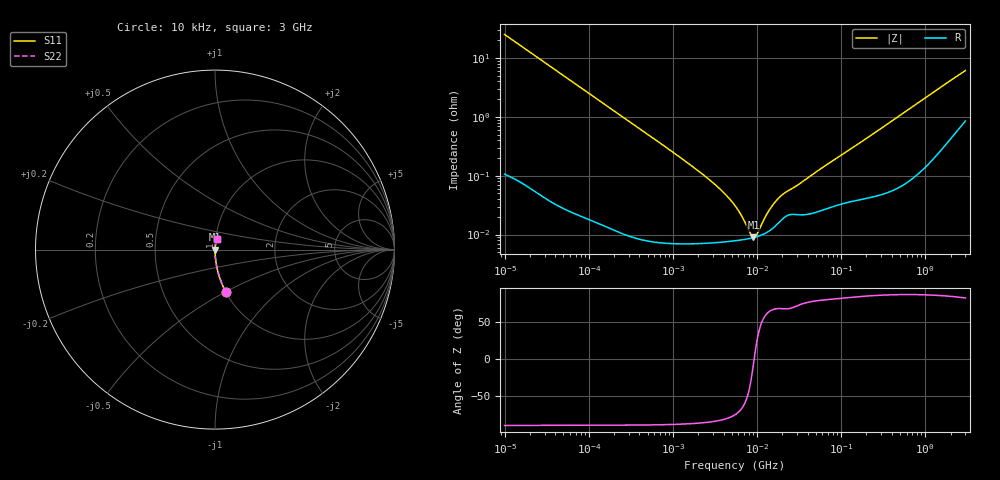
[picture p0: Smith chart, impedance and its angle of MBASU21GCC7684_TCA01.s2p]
! MBASU21GCC7684_TCA01  S-PARAMETER MODEL  ( Standard Model )
! Model Generated by TAIYO YUDEN Corporation (http://www.ty-top.com)
! Version 1.0
! TAIYO YUDEN Control No. 220601
! Copyright(c) 2014 TAIYO YUDEN CO.,LTD. All Rights Reserved.
! Product Description (link to TY-COMPAS)
! https://ds.yuden.co.jp/TYCOMPAS/or/detail?pn=MBASU21GCC7684KTCA01&u=M
! Products Name : Multilayer Ceramic Capacitors
! Characteristics :
!  Capacitance : 0.68 [uF] , Rated Voltage : 50 [V] , TCC : X7S
!  Case Size : 2.0 x 1.25 / 0.079 x 0.049 [mm/inch] , Thickness : 1.25 / 0.049 [mm/inch]
!  (Conditions: Temperature = 25 [degC] , DC Bias Voltage = 0 [V])
! External Node Assignments :
!  1  o---| |---o  2
! GND o---------o GND
! Frequency Range : 10kHz  -  3GHz  [ 401 STEP ]
# MHZ S RI R 50
! Freq[MHz].  S11 Real  S11 Imag  S21 Real  S21 Imag  S12 Real  S12 Imag  S22 Real  S22 Imag
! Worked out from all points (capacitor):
!   401 points, 10 kHz to 3 GHz, reference 50 ohm
!   read as one part in series: C = 631 nF near 10.65 kHz
!   lowest |Z| = 8.95 mohm at 9.071 MHz (marker M1)
!   series resonance near 9.261 MHz, so ESL is about 470 pH
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0.01  0.0605 -0.2364  0.9395 0.2364  0.9395 0.2364  0.0605 -0.2364
0.02575  0.01 -0.0971  0.99 0.0971  0.99 0.0971  0.01 -0.0971
0.082683  0.00114 -0.0306  0.9989 0.0306  0.9989 0.0306  0.00114 -0.0306
0.683653  8.65e-05 -0.00371  0.9999 0.00371  0.9999 0.00371  8.65e-05 -0.00371
1.601553  7.18e-05 -0.00154  0.9999 0.00154  0.9999 0.00154  7.18e-05 -0.00154
2.737278  7.24e-05 -0.000846  0.9999 0.000846  0.9999 0.000846  7.24e-05 -0.000846
4.124064  7.54e-05 -0.000492  0.9999 0.000492  0.9999 0.000492  7.54e-05 -0.000492
5.477226  7.86e-05 -0.0003  0.9999 0.0003  0.9999 0.0003  7.86e-05 -0.0003
6.617858  8.14e-05 -0.000187  0.9999 0.000187  0.9999 0.000187  8.14e-05 -0.000187
8.252149  8.6e-05 -6.33e-05  0.9999 6.33e-05  0.9999 6.33e-05  8.6e-05 -6.33e-05
9.070798  8.87e-05 -1.13e-05  0.9999 1.13e-05  0.9999 1.13e-05  8.87e-05 -1.13e-05
9.6612  9.09e-05 2.32e-05  0.9999 -2.32e-05  0.9999 -2.32e-05  9.09e-05 2.32e-05
10.29003  9.34e-05 5.8e-05  0.9999 -5.8e-05  0.9999 -5.8e-05  9.34e-05 5.8e-05
13.66633  0.000113 0.000219  0.9999 -0.000219  0.9999 -0.000219  0.000113 0.000219
15.50326  0.000129 0.000295  0.9999 -0.000295  0.9999 -0.000295  0.000129 0.000295
18.15044  0.000159 0.000388  0.9998 -0.000388  0.9998 -0.000388  0.000159 0.000388
21.24962  0.000197 0.00047  0.9998 -0.00047  0.9998 -0.00047  0.000197 0.00047
30.05882  0.000219 0.00065  0.9998 -0.00065  0.9998 -0.00065  0.000219 0.00065
45.28751  0.00023 0.00102  0.9998 -0.00102  0.9998 -0.00102  0.00023 0.00102
374.4521  0.000593 0.00794  0.9994 -0.00794  0.9994 -0.00794  0.000593 0.00794
1755.269  0.00469 0.0362  0.9953 -0.0362  0.9953 -0.0362  0.00469 0.0362
3000  0.012 0.0594  0.988 -0.0594  0.988 -0.0594  0.012 0.0594
